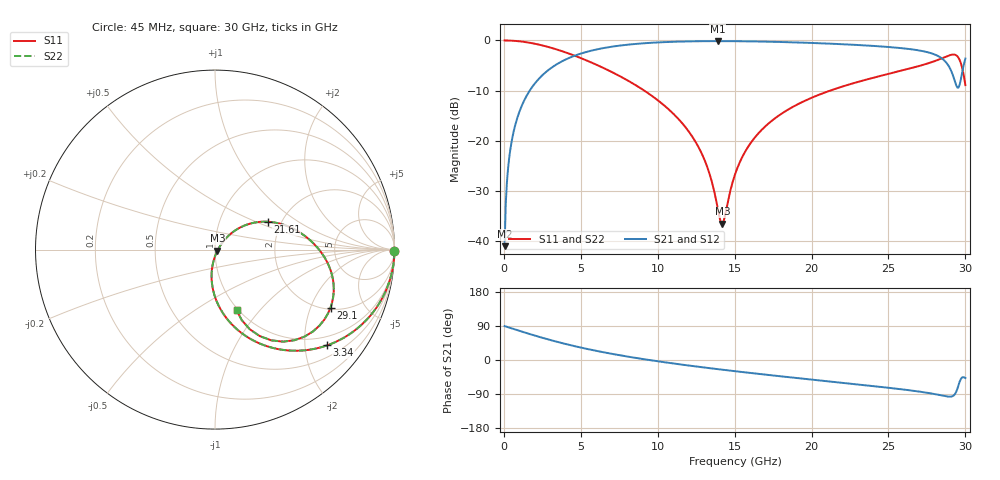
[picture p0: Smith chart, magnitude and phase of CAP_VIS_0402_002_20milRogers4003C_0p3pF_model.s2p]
! S-parameter model data by Modelithics Inc.  support@modelithics.com  813-866-6335  Tampa FL USA
! S-Parameter data specifications:
! Substrate: 20-mil Rogers 4003C, substrate thickness, H=0.508mm, Dielectric constant, Er=3.75
! PCB Mounting Pad Footprint: Pad width, PadW=0.50mm , Pad length, PadL=0.50mm , Pad gap, PadG (edge-to-edge)=0.40mm , Reference planes=1.4mm apart
! Created Wed Nov 18 12:41:42 2015
# hz S ma R 50
! 2 Port Network Data from SP1.SP block
! freq  magS11  angS11  magS21  angS21  magS12  angS12  magS22  angS22
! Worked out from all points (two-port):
!   401 points, 45 MHz to 30 GHz, reference 50 ohm
!   highest |S21| = -0.13 dB at 13.9 GHz (marker M1); lowest = -41.1 dB at 45 MHz (marker M2)
!   |S21| within 3 dB of the highest: 4.527 GHz to 28.23 GHz (23.71 GHz wide, 145 % of centre)
!   lowest |S11| = -36.6 dB at 14.2 GHz (marker M3), VSWR 1.03, Z = 51.4 - j0.594 ohm
!   |S11| at or under -10 dB: 9.113 GHz to 21.23 GHz (12.11 GHz wide, 79.9 % of centre)
!   |S22| runs from -36.6 to 0.0 dB; largest |S21 - S12| = 0
!   S11 on the Smith chart (normalised r, x): 45 MHz: open; 3.34 GHz: 0.76, -2.51; 21.61 GHz: 1.70, +0.59; 29.1 GHz: 2.08, -2.79; 30 GHz: 0.98, -0.76
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4.5e7  1 -0.6  0.008805 89.4  0.008805 89.4  1 -0.6
3.4455e8  0.9977 -4.5  0.0673 85.5  0.0673 85.5  0.9977 -4.5
8.687625e8  0.9856 -11.2  0.1681 78.7  0.1681 78.7  0.9856 -11.2
1.8423e9  0.9384 -23.4  0.3437 66.5  0.3437 66.5  0.9384 -23.4
3.34005e9  0.8213 -40.5  0.5664 49.2  0.5664 49.2  0.8213 -40.5
5.062462e9  0.6606 -57.2  0.7443 32.2  0.7443 32.2  0.6606 -57.2
7.458862e9  0.4461 -75.8  0.8857 13.1  0.8857 13.1  0.4461 -75.8
1.007992e10  0.2474 -91.2  0.9571 -3.8  0.9571 -3.8  0.2474 -91.2
1.26261e10  0.08736 -98.8  0.9823 -17.8  0.9823 -17.8  0.08736 -98.8
1.337498e10  0.04609 -93.7  0.9845 -21.6  0.9845 -21.6  0.04609 -93.7
1.389919e10  0.02108 -70.7  0.9849 -24.2  0.9849 -24.2  0.02108 -70.7
1.419874e10  0.01473 -23.1  0.9848 -25.6  0.9848 -25.6  0.01473 -23.1
1.50225e10  0.04576 40.9  0.9833 -29.6  0.9833 -29.6  0.04576 40.9
1.577138e10  0.08169 45.8  0.9805 -33.0  0.9805 -33.0  0.08169 45.8
1.68198e10  0.1307 44.9  0.9745 -37.8  0.9745 -37.8  0.1307 44.9
2.003996e10  0.269 34.1  0.9439 -51.9  0.9439 -51.9  0.269 34.1
2.16126e10  0.3312 28.0  0.923 -58.6  0.923 -58.6  0.3312 28.0
2.505742e10  0.4655 13.3  0.8591 -73.6  0.8591 -73.6  0.4655 13.3
2.782826e10  0.6086 -3.6  0.7407 -88.6  0.7407 -88.6  0.6086 -3.6
2.910135e10  0.7202 -26.6  0.4861 -96.3  0.4861 -96.3  0.7202 -26.6
2.955068e10  0.6719 -48.7  0.3381 -66.7  0.3381 -66.7  0.6719 -48.7
3e10  0.3574 -70.4  0.6597 -47.7  0.6597 -47.7  0.3574 -70.4
